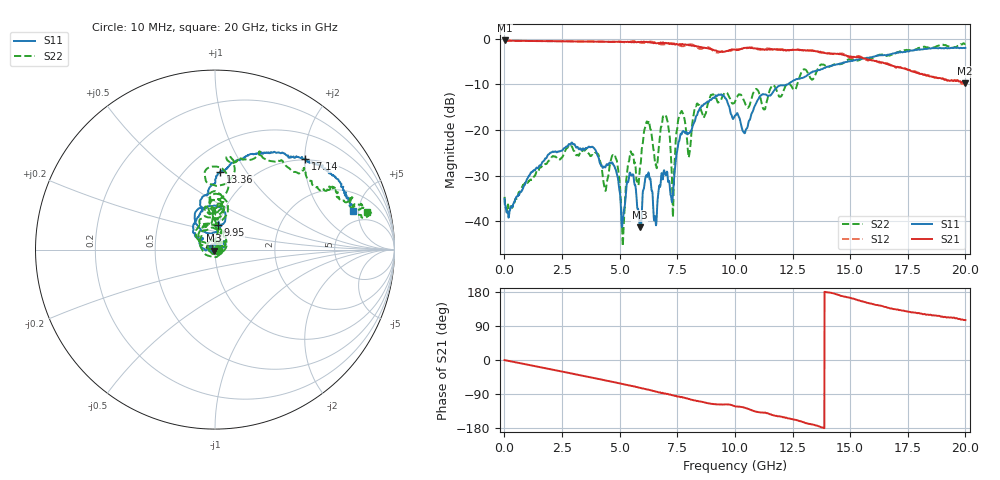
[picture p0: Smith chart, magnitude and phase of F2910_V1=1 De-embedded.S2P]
! Integrated Device Technology
! Corporate Headquarters
! 6024 Silver Creek Valley Road
! San Jose, CA 95138  USA
! Phone:  1-408-284-8200
! Toll Free:  1-800-223-1366
! Webpage:  http://www.idt.com/
! Timing and RF Division
! 515 Groton Road, Suite 102
! Westford, MA 01886-6024
! Device:  F2910
! Description: Constant Impedance K|Z| SPST RF Switch
! Frequency:  0.030 - 8.000 GMHz
! Package:  2x2 mm DFN Plastic Package: 8 pin
! Ports:  2 RF, 2 DC
!  Pin  1  = NC
!  Pin  2  = GND
!  Pin  3  = GND
!  Pin  4  = NC
!  Pin  5  = RF1  = Port 1
!  Pin  6  = VDD
!  Pin  7  = V1
!  Pin  8  = RF2  = Port 2
! Voltage:  Vcc  =  +3.30 Volts
! Current:  Icc  = 370  uA
! State:  ON
! V1:  Logic HIGH
! Data:  The device was measured on the F2910 evaluation board which has
!  individual transmission lines to the RF pins.  Data was collected
!  using a calibrated network analyzer.  The input lines were
!  modeled using Automatic Fixture Removal (AFR) from Keysight.
!  The reference plane is at the package pin.
!  data was collected with the high frequency option using capacitors
!  on Vcc and V1 pins.
! Misc:
!  Action Tracker AT0436
! Date Measured:  2018-12-14
! Date:  2018-12-14  MJV
! Note:
!  Integrated Device Technology supplies this data as a sample of measured
!  data at the evaluation board for this product.  Your particular data for this
!  product may vary.
!  Data was taken at 25 degrees C.
!  Integrated Device Technology reserves the right to change this data at anytime.
# Hz S dB R 50
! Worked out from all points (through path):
!   2000 points, 10 MHz to 20 GHz, reference 50 ohm
!   highest |S21| = -0.36 dB at 10 MHz (marker M1); lowest = -9.8 dB at 19.99 GHz (marker M2)
!   group delay of S21, straight-line fit = 36.6 ps
!   lowest |S11| = -41.4 dB at 5.87 GHz (marker M3), VSWR 1.02, Z = 49.5 - j0.66 ohm
!   |S11| at or under -10 dB: start of sweep to 12.3 GHz
!   |S22| runs from -45.5 to -1.0 dB; largest |S21 - S12| = 0.052
!   S11 on the Smith chart (normalised r, x): 10 MHz: 1.03, -0.01; 9.95 GHz: 0.99, +0.27; 13.36 GHz: 0.72, +0.76; 17.14 GHz: 0.98, +2.02; 20 GHz: 3.67, +4.31
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1e7  -35.16 -10.3  -0.36 -0.3  -0.37 -0.3  -34.68 -10.9
3.35e9  -24.47 33.3  -0.56 -40.9  -0.56 -41.0  -24.96 45.9
4.38e9  -28.20 30.2  -0.63 -53.8  -0.65 -53.7  -33.38 38.8
4.79e9  -28.21 10.1  -0.67 -58.8  -0.62 -59.3  -25.43 66.4
5.14e9  -39.90 28.2  -0.66 -63.6  -0.72 -63.2  -45.51 70.7
5.51e9  -29.99 42.8  -0.75 -68.2  -0.58 -69.5  -25.15 120.4
5.87e9  -41.39 -128.5  -0.72 -73.3  -0.76 -72.0  -28.75 -26.3
6.19e9  -30.10 74.2  -0.66 -77.9  -0.75 -80.1  -18.17 99.1
6.68e9  -33.77 -146.2  -0.92 -85.2  -1.06 -83.6  -24.52 6.5
7e9  -29.92 139.0  -0.90 -88.8  -1.16 -90.9  -16.89 117.4
7.31e9  -34.27 167.8  -1.18 -93.1  -0.99 -93.2  -39.17 117.4
7.62e9  -21.44 165.8  -1.13 -97.5  -1.51 -95.9  -16.46 104.9
8.01e9  -20.73 137.5  -1.43 -102.8  -1.26 -104.3  -25.78 114.7
8.57e9  -14.65 129.0  -1.86 -110.5  -2.17 -111.8  -16.12 120.3
9.95e9  -17.34 84.0  -2.35 -120.9  -2.39 -121.9  -14.15 84.2
1.001e10  -16.84 87.5  -2.35 -122.1  -2.33 -123.1  -13.72 80.7
1.334e10  -7.37 86.8  -2.63 -169.8  -2.50 -170.2  -8.98 89.4
1.336e10  -7.26 86.3  -2.58 -170.1  -2.52 -170.3  -8.96 87.8
1.667e10  -3.54 50.6  -5.69 137.6  -5.53 137.8  -3.64 35.0
1.714e10  -2.93 45.1  -6.28 131.7  -6.26 130.4  -2.78 27.8
1.999e10  -2.00 15.5  -9.76 105.3  -10.10 104.3  -1.18 13.9
2e10  -1.96 15.5  -9.76 105.3  -10.09 104.0  -1.17 13.9
